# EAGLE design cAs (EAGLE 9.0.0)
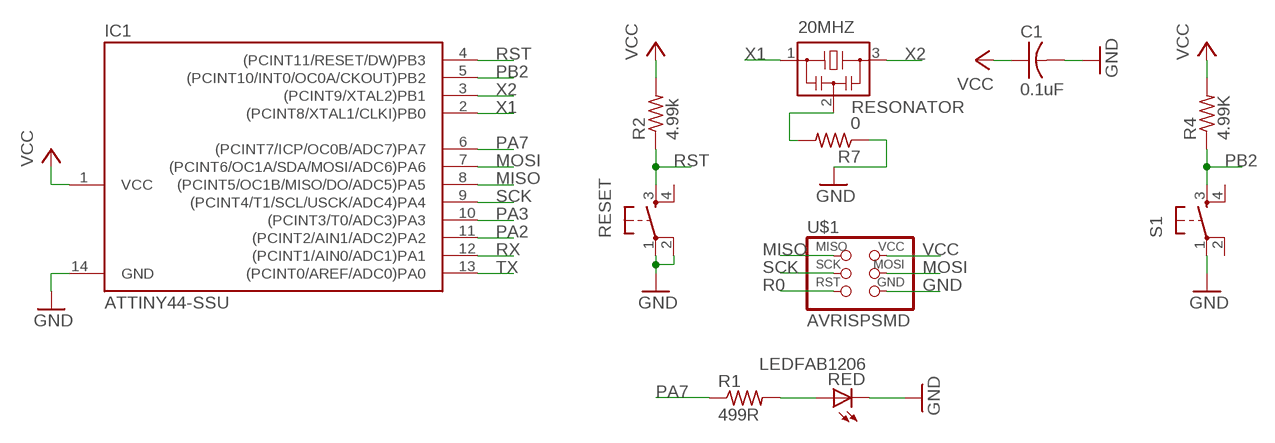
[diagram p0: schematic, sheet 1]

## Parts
20MHZ  RESONATOR  [EFOBM]
C1  0.1uF  CAP-US1206K  [C1206K]
IC1  ATTINY44-SSU  [SOIC14]
R1  499R  RES-US1206FAB  [R1206FAB]
R2  4.99k  RES-US1206FAB  [R1206FAB]
R4  4.99K  RES-US1206FAB  [R1206FAB]
R7  0  RES-US1206FAB  [R1206FAB]
RED  LEDFAB1206  [LED1206FAB]
RESET  6MM_SWITCH6MM_SWITCH  [6MM_SWITCH]
S1  6MM_SWITCH6MM_SWITCH  [6MM_SWITCH]
U$1  AVRISPSMD  [2X03SMD]

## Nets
GND: C1.2 IC1.14(GND) R7.1 RED.2(C) RESET.1(P) RESET.2(P1) S1.1(P) U$1.6(GND)
MISO: IC1.8((PCINT5/OC1B/MISO/DO/ADC5)PA5) U$1.1(MISO)
MOSI: IC1.7((PCINT6/OC1A/SDA/MOSI/ADC6)PA6) U$1.4(MOSI)
N$1: R1.2 RED.1(A)
N$2: 20MHZ.2 R7.2
PA2: IC1.11((PCINT2/AIN1/ADC2)PA2)
PA3: IC1.10((PCINT3/T0/ADC3)PA3)
PA7: IC1.6((PCINT7/ICP/OC0B/ADC7)PA7) R1.1
PB2: IC1.5((PCINT10/INT0/OC0A/CKOUT)PB2) R4.1 S1.3(S)
R0: U$1.5(RST)
RST: IC1.4((PCINT11/RESET/DW)PB3) R2.1 RESET.3(S)
RX: IC1.12((PCINT1/AIN0/ADC1)PA1)
SCK: IC1.9((PCINT4/T1/SCL/USCK/ADC4)PA4) U$1.3(SCK)
TX: IC1.13((PCINT0/AREF/ADC0)PA0)
VCC: C1.1 IC1.1(VCC) R2.2 R4.2 U$1.2(VCC)
X1: 20MHZ.1 IC1.2((PCINT8/XTAL1/CLKI)PB0)
X2: 20MHZ.3 IC1.3((PCINT9/XTAL2)PB1)
Unconnected: RESET.4(S1) S1.2(P1) S1.4(S1)

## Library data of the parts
20MHZ = fab:RESONATOR
C1 = fab:CAP-US
IC1 = fab:ATTINY44
R1 R2 R4 R7 = fab:RES-US: Resistor (US Symbol)
RED = fab:LED: LED
RESET S1 = fab:6MM_SWITCH: OMRON SWITCH
U$1 = fab:AVRISP

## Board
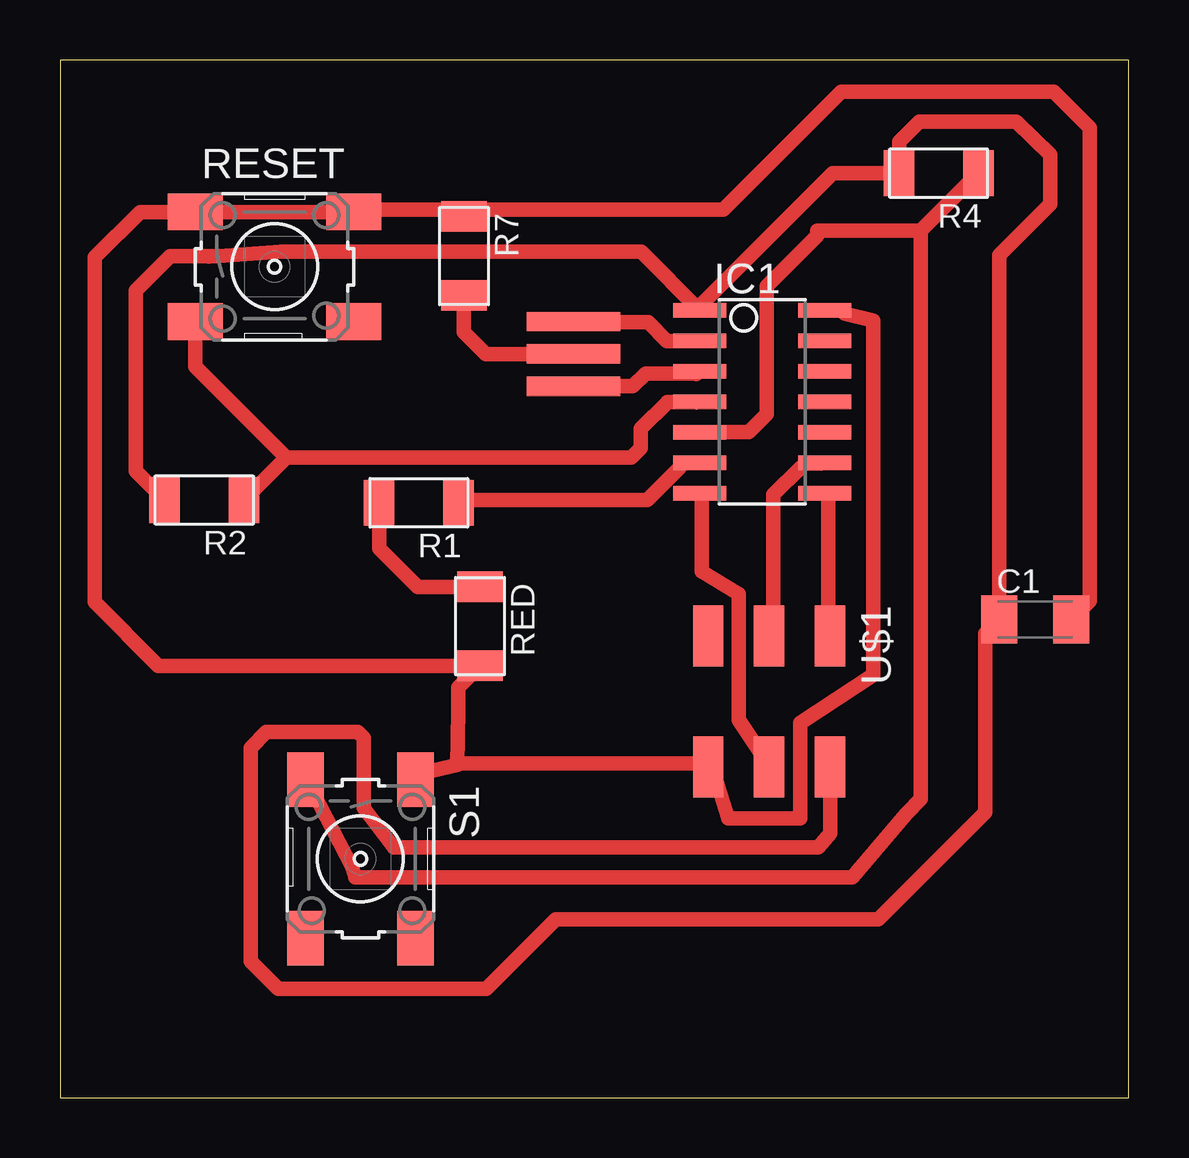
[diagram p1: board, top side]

Size 44.54 x 43.27 mm. Coordinates in mm from the lower left corner, seen from the top.
Outline: 0,0 44.54,0 44.54,43.27 0,43.27 0,0
Copper layers (1*16): Top 0.035mm / dielectric 1.5mm / Bottom 0.035mm
Design rules "default": minimum track width 10mil, minimum drill 24mil, track to track 8mil, track to pad 8mil, pad to pad 8mil, via to via 8mil, smd to smd 8mil, copper to edge 40mil, drill to drill 8mil, minimum pad ring 10mil, minimum via ring 8mil, stop-mask expansion 4mil, vias tented up to drill 0mil, thermal gap 10mil

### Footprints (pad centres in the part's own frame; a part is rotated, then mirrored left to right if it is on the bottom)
EFOBM = smd 0.8 x 3.9: 1 -1.35,0; 2 0,0; 3 1.35,0
C1206K = smd 1.5 x 2: 1 -1.5,0; 2 1.5,0
SOIC14 = smd 0.61 x 2.21: 1 -3.81,-2.603; 2 -2.54,-2.603; 3 -1.27,-2.603; 4 0,-2.603; 5 1.27,-2.603; 6 2.54,-2.603; 7 3.81,-2.603; 8 3.81,2.603; 9 2.54,2.603; 10 1.27,2.603; 11 0,2.603; 12 -1.27,2.603; 13 -2.54,2.603; 14 -3.81,2.603
R1206FAB = smd 1.27 x 1.905: 1 -1.651,0; 2 1.651,0
LED1206FAB = smd 1.27 x 1.905: 1 -1.651,0; 2 1.651,0
6MM_SWITCH = smd 2.286 x 1.524: 1 -3.302,2.286; 2 3.302,2.286; 3 -3.302,-2.286; 4 3.302,-2.286
2X03SMD = smd 2.54 x 1.27: 1 -2.54,2.54; 2 2.92,2.54; 3 -2.54,0; 4 2.92,0; 5 -2.54,-2.54; 6 2.92,-2.54

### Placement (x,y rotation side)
20MHZ  21.4,31.02 270 top
C1  40.63,19.94 0 top
IC1  29.26,29.02 270 top
R1  14.95,24.81 180 top
R2  6.01,24.93 180 top
R4  36.61,38.55 180 top
R7  16.83,35.1 270 top
RED  17.5,19.67 270 top
RESET  8.94,34.65 0 top
S1  12.52,9.97 270 top
U$1  29.55,16.72 270 top

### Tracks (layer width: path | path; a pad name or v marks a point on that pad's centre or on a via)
GND
  Top 0.254: 12.8,37.03 12.34,36.58 RESET.2 | 16.69,37.03 R7.1 16.92,37.03 | 31.77,32.92 IC1.14 32,32.69 32.69,32.69 | 27.2,13.72 U$1.6 26.98,13.95 | 14.86,13.49 S1.1
  Top 0.61: 12.8,37.03 16.69,37.03 | 16.92,37.03 27.63,37.03 32.55,41.95 41.4,41.95 42.9,40.45 42.9,20.71 C1.2 | 27.2,13.72 27.85,11.67 30.84,11.67 30.84,15.64 33.88,17.63 33.88,32.4 32.69,32.69 | 16.55,13.88 16.6,16.13 16.6,17.12 RED.2 4.1,18.02 1.44,20.67 1.44,35.04 3.34,36.94 RESET.1 RESET.2 | 14.86,13.49 16.55,13.88 | 26.98,13.95 16.69,13.95 16.55,13.88
MISO
  Top 0.254: 32,25.15 IC1.8 | 32,19.43 U$1.1
  Top 0.61: 32,19.43 32,25.15
MOSI
  Top 0.254: 26.75,25.15 IC1.7 | 29.49,13.95 U$1.4
  Top 0.61: 26.75,25.15 26.75,21.95 28.27,21.02 28.27,15.76 29.49,13.95
N$1
  Top 0.254: 13.26,24.69 R1.2
  Top 0.61: R1.2 13.3,22.9 14.9,21.3 17.48,21.3 RED.1
N$2
  Top 0.254: 16.92,33.83 R7.2
  Top 0.61: 20MHZ.2 17.73,31.02 16.83,31.92 R7.2
PA7
  Top 0.254: 25.83,26.29 26.52,26.29 IC1.6 | 16.69,24.92 R1.1
  Top 0.61: 16.69,24.92 24.46,24.92 25.83,26.29
PB2
  Top 0.254: 10.29,13.26 S1.3
  Top 0.61: 10.29,13.26 12.19,9.61 12.3,9.2 33,9.2 35.25,11.85 35.86,12.46 35.86,36.15 | IC1.5 28.7,27.75 29.45,28.5 29.45,33.85 31.55,35.95 31.55,36.15 35.86,36.15 | 35.86,36.15 R4.1
RST
  Top 0.254: 5.49,31.77 RESET.3 | 26.52,28.8 IC1.4
  Top 0.61: 25.3,29 26.64,29 IC1.4 25.32,29.02 24.2,27.9 24.2,27.1 23.8,26.7 9.43,26.7 | 9.43,26.7 R2.1 | RESET.3 5.64,30.49 9.43,26.7
SCK
  Top 0.254: 30.86,26.29 31.77,26.29 IC1.9 | 29.72,19.43 U$1.3
  Top 0.61: 30.86,26.29 29.72,25.15 29.72,19.43
VCC
  Top 0.254: 32.18,13.99 U$1.2 | 26.52,32.92 26.55,32.9 IC1.1
  Top 0.61: 6.6,35.1 9.19,35.28 24.21,35.28 IC1.1 | 6.6,35.1 6.2,35.08 | 6.6,35.1 4.6,35.1 3.15,33.65 3.15,26.14 R2.2 | 26.55,32.9 32.2,38.55 R4.2 34.96,39.86 35.8,40.7 39.85,40.7 41.27,39.33 41.27,37.27 39.13,35.13 C1.1 38.55,19.36 38.55,11.9 34.1,7.45 20.65,7.45 17.75,4.55 9.1,4.55 7.95,5.7 7.95,14.6 8.6,15.25 12.4,15.25 12.65,15 12.65,12.1 13.9,10.45 31.6,10.45 32.09,11.04 U$1.2
X1
  Top 0.61: IC1.2 25.29,31.56 24.5,32.35 21.42,32.35 20MHZ.1
X2
  Top 0.254: 26.52,30.18 IC1.3
  Top 0.61: 20MHZ.3 23.87,29.67 24.4,30.2 26.49,30.2 26.52,30.18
